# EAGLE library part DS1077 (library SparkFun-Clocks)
Maxim DS1077 - I2C Real-time clock (RTC) The DS1077 is a dual-output, programmable, fixed-frequency oscillator requiring no external components for operation. The DS1077 can be used as a processor-controlled frequency synthesizer or as a standalone oscillator. The DS1077 features a 2-wire serial interface that allows in-circuit on-the-fly programming of the programmable prescalers (P0 & P1) and divider (N) with the desired values being stored in NV (EEPROM) memory. SparkFun Products: Real Time Clock Module (BOB-00099) Datasheet
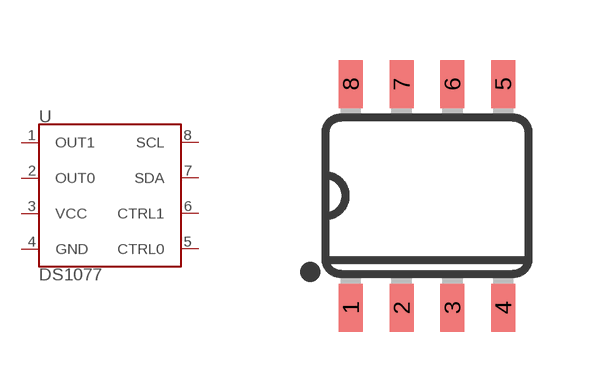
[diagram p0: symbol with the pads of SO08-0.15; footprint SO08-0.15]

Designator prefix U

## DS1077U (PROD_ID: IC-09075)  [SO08-0.15]
1  OUT1
2  OUT0
3  VCC
4  GND
5  CTRL0
6  CTRL1
7  SDA
8  SCL

## Footprint SO08-0.15 (pad centres in mm)
8-Pin SOIC 150mil 0.154" (3.9mm) width. Fits JEDEC packages (narrow SOIC-8). Used by DS1077 and DS1307 programmable oscillators
smd 0.6 x 1.2: 1 -1.905,-2.8; 2 -0.635,-2.8; 3 0.635,-2.8; 4 1.905,-2.8; 5 1.905,2.8; 6 0.635,2.8; 7 -0.635,2.8; 8 -1.905,2.8

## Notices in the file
Licensing: Creative Commons ShareAlike 4.0 International - https://creativecommons.org/licenses/by-sa/4.0
